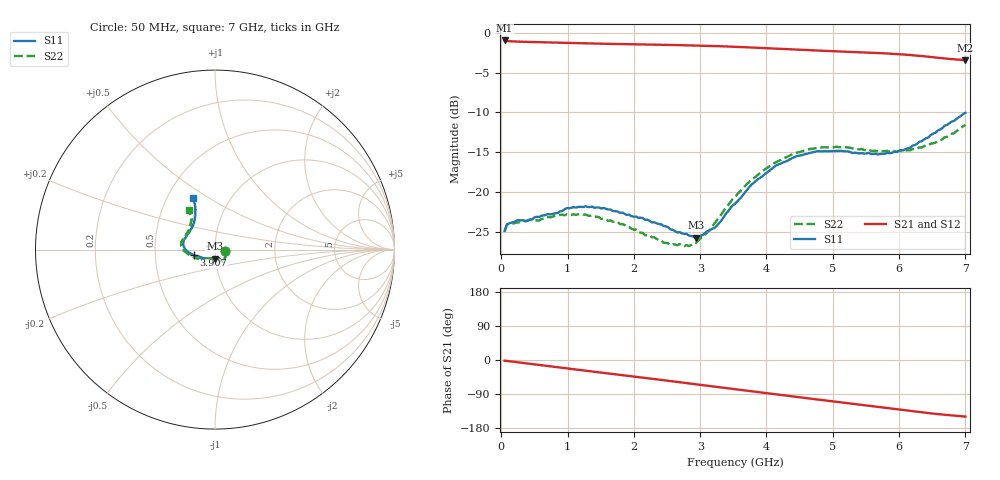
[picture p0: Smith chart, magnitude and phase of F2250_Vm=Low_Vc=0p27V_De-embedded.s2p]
! Integrated Device Technology
! Corporate Headquarters
! 6024 Silver Creek Valley Road
! San Jose, CA 95138  USA
! Phone:  1-408-284-8200
! Toll Free:  1-800-223-1366
! Webpage:  http://www.idt.com/
! Timing and RF Division
! 515 Groton Road, Suite 102
! Westford, MA 01886-6024
! Device:  F2250
! Description: Voltage Variable RF Attenuator
! Frequency:  50.0 -  6000.00 MHz
! Package:  3x3 mm Thin QFN Plastic Package: 16 pin
! Ports:  2 RF, 3 DC
!  Pin  1  = GND
!  Pin  2  = NC
!  Pin  3  = RF1  = Port 1
!  Pin  4  = NC
!  Pin  5  = GND
!  Pin  6  = GND
!  Pin  7  = GND
!  Pin  8  = GND
!  Pin  9  = NC
!  Pin 10  = RF2  = Port 2
!  Pin 11  = NC
!  Pin 12  = GND
!  Pin 13  = GND
!  Pin 14  = VCNTRL
!  Pin 15  = VDD
!  Pin 16  = VMODE
! Vcntrl:  0.270 Volts
! Vmode:  +0.000 Volts
! Vdd:  +3.30  Volts
! Current:  1.109 mA
! Data:  The device was measured on a the F2250 evaluation board which has
!  individual transmission lines to the RF pins.  Data was collected
!  using a calibrated network analyzer.  The evaluation board was
!  de-embedded using a TRL calibration technique.
!  The reference plane is the edge of the package pin.
! Misc:  SN 10
!  Action Tracker AT0258
! Date Measured:  2014-11-26
! Date:  2015-10-15  MJV
! Note:
!  Integrated Device Technology supplies this data as a sample of measured
!  data at the package pin for this product.  Your particular data for this
!  product may vary.
!  Data was taken at 25 degrees C.
!  Integrated Device Technology reserves the right to change this data at anytime.
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# GHz S dB R 50
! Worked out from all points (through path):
!   201 points, 50 MHz to 7 GHz, reference 50 ohm
!   highest |S21| = -0.94 dB at 50 MHz (marker M1); lowest = -3.4 dB at 7 GHz (marker M2)
!   group delay of S21, straight-line fit = 60 ps
!   lowest |S11| = -25.8 dB at 2.934 GHz (marker M3), VSWR 1.11, Z = 49.6 - j5.12 ohm
!   |S11| at or under -10 dB: start of sweep to end of sweep
!   |S22| runs from -26.8 to -11.6 dB; largest |S21 - S12| = 0.00032
!   S11 on the Smith chart (normalised r, x): 50 MHz: 1.12, -0.02; 3.907 GHz: 0.79, -0.05; 7 GHz: 0.67, +0.43
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0.05  -24.89 -9.5  -0.94 -1.8  -0.94 -1.8  -25.00 -9.9
0.08475  -24.07 -9.4  -1.01 -2.5  -1.01 -2.5  -24.13 -9.2
0.15425  -23.85 -11.7  -1.05 -4.0  -1.05 -4.0  -23.89 -11.0
0.57125  -23.15 -29.6  -1.16 -13.1  -1.16 -13.1  -23.61 -30.1
0.884  -22.45 -45.3  -1.22 -19.9  -1.22 -19.9  -22.88 -46.5
1.2315  -21.91 -55.4  -1.30 -27.4  -1.30 -27.4  -22.88 -59.3
1.75275  -22.46 -62.1  -1.39 -38.4  -1.39 -38.4  -23.75 -66.4
2.37825  -24.05 -62.9  -1.48 -51.8  -1.48 -51.8  -26.05 -68.1
2.552  -24.72 -67.0  -1.51 -55.6  -1.50 -55.6  -26.69 -73.7
2.83  -25.50 -82.2  -1.56 -61.7  -1.56 -61.7  -26.82 -92.7
2.93425  -25.78 -91.1  -1.58 -64.0  -1.58 -64.0  -26.44 -101.5
3.21225  -24.55 -120.6  -1.64 -70.2  -1.64 -70.2  -24.01 -127.3
3.525  -21.49 -147.3  -1.74 -77.1  -1.74 -77.1  -20.63 -146.1
3.76825  -19.13 -160.6  -1.83 -82.5  -1.83 -82.5  -18.49 -156.5
3.90725  -18.21 -164.9  -1.88 -85.5  -1.88 -85.5  -17.60 -162.6
4.1505  -16.65 -173.2  -1.98 -90.8  -1.98 -90.8  -16.22 -171.2
4.7065  -15.00 172.6  -2.19 -102.8  -2.19 -102.8  -14.56 175.7
5.15825  -14.86 161.9  -2.35 -112.6  -2.35 -112.6  -14.32 166.6
5.85325  -15.13 138.7  -2.60 -127.5  -2.60 -127.5  -14.94 151.5
6.166  -14.44 127.8  -2.77 -134.3  -2.77 -134.3  -14.76 142.7
6.444  -13.13 119.5  -2.98 -140.1  -2.98 -140.1  -14.14 133.3
7  -10.05 113.2  -3.42 -149.4  -3.42 -149.4  -11.57 123.8
